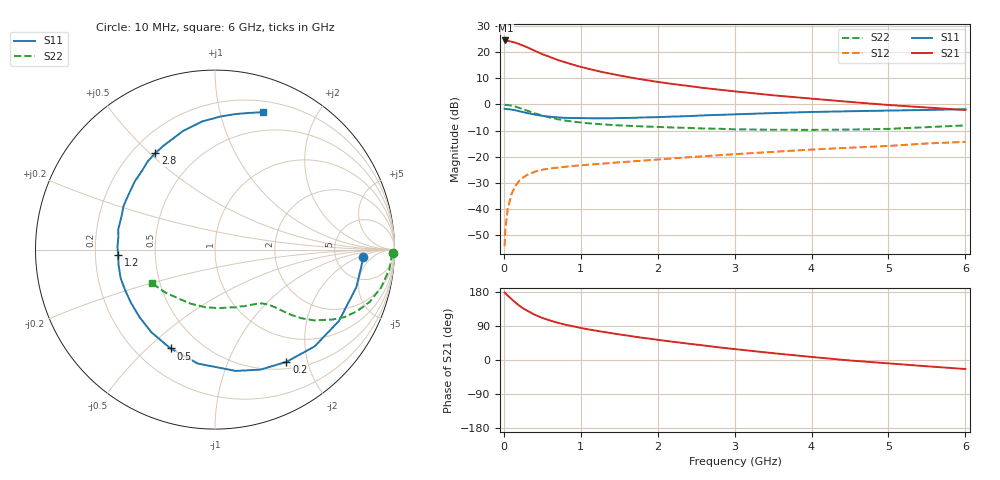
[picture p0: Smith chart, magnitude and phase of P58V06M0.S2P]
! SIEMENS Small Signal Semiconductors
! BFP183
! Si NPN RF Bipolar Junction Transistor in SOT143
! VCE = 8 V  IC = 6 mA
! Common Emitter S-Parameters:  March  1996
# GHz  S  MA  R  50
!  f  S11  S21  S12  S22
! GHz  MAG  ANG  MAG  ANG  MAG  ANG  MAG  ANG
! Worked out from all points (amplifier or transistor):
!   36 points, 10 MHz to 6 GHz, reference 50 ohm
!   highest |S21| = 24.6 dB at 20 MHz (marker M1)
!   |S21| within 3 dB of that: start of sweep to 330.3 MHz
!   unconditionally stable (mu >= 1): 1.554 GHz to 5.705 GHz
!   at 250 MHz: K = 0.22, MSG = 25.3 dB, |S12| = -28.1 dB
!   at 1.4 GHz: K = 0.95, MSG = 17.1 dB, |S12| = -22.5 dB
!   at 6 GHz: K = 0.95, MSG = 6.1 dB, |S12| = -14.4 dB
!   lowest NFmin = 1.20 dB at 450 MHz
!   S11 on the Smith chart (normalised r, x): 10 MHz: 10, -3; 200 MHz: 0.60, -1.66; 500 MHz: 0.34, -0.59; 1.2 GHz: 0.30, -0.03; 2.8 GHz: 0.29, +0.52; 6 GHz: 0.31, +1.36
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0.01  0.8264 -3.0  16.92 177.9  0.0019 87.8  0.9913 -1.2
0.02  0.8211 -6.4  16.98 176.3  0.004 84.7  0.9844 -2.6
0.05  0.8144 -15.1  16.7 170.1  0.0098 82.2  0.9776 -6.5
0.1  0.7968 -30.0  16.07 160.7  0.0191 73.9  0.9496 -12.8
0.15  0.7739 -44.2  15.36 151.8  0.0272 66.7  0.9097 -18.7
0.2  0.7414 -57.5  14.48 143.7  0.0342 62.3  0.8627 -23.4
0.25  0.7152 -69.2  13.5 136.4  0.0394 56.7  0.814 -27.5
0.3  0.6859 -80.3  12.6 130.5  0.0442 52.5  0.7629 -30.7
0.4  0.642 -98.6  10.78 119.6  0.051 45.8  0.6795 -35.5
0.5  0.604 -114.2  9.261 111.1  0.0558 41.6  0.6138 -38.5
0.6  0.5814 -127.5  8.178 104.2  0.0591 38.5  0.5617 -40.5
0.7  0.5643 -138.2  7.169 98.4  0.0613 36.7  0.5214 -41.8
0.8  0.5541 -147.7  6.453 93.2  0.0636 35.1  0.4918 -42.8
1.1  0.5442 -170.4  4.854 80.7  0.0699 33.4  0.4355 -45.3
1.2  0.5417 -176.6  4.47 77.3  0.0716 32.9  0.4247 -46.2
1.7  0.5556 158.4  3.194 61.6  0.0815 33.6  0.3849 -51.7
2.2  0.5861 139.9  2.47 48.1  0.0923 33.8  0.3614 -59.0
2.8  0.6319 121.8  1.925 33.2  0.1062 32.7  0.3417 -70.3
3.5  0.6844 105.1  1.503 18.0  0.1232 30.9  0.3269 -86.1
4.5  0.7421 87.6  1.12 -1.3  0.1479 26.0  0.3299 -113.7
5.5  0.7848 76.0  0.875 -16.6  0.1783 21.0  0.3667 -139.6
6  0.8106 70.8  0.784 -23.8  0.1915 17.1  0.3965 -151.6
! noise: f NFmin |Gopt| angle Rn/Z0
0.45  1.2  0.21  41  0.24
0.9  1.25  0.24  101  0.21
1.8  2  0.32  175  0.14
